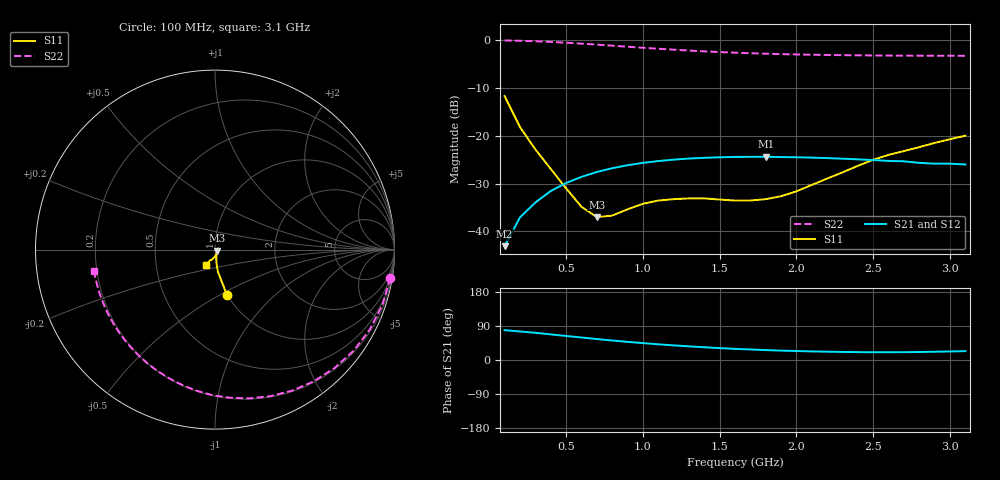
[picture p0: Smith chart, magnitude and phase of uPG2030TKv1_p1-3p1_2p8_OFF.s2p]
! NEC Compound Semiconductor Devices Ltd.
! 21.January 2005
! uPG2030TK
! GaAs MMIC (0.1 - 3.1GHz SPDT switch)
! Vcont1=0v Vcont2=2.8v / IN-OUT1 ( OFF )
! OUT2:50ohm termination
#  GHz  S  MA  R  50
!  f  S11  S21  S12  S22
!  GHz  MAG  ANG  MAG  ANG  MAG  ANG  MAG  ANG
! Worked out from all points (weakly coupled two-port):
!   31 points, 100 MHz to 3.1 GHz, reference 50 ohm
!   highest |S21| = -24.41 dB at 1.8 GHz (marker M1); lowest = -43.1 dB at 100 MHz (marker M2)
!   lowest |S11| = -37.0 dB at 700 MHz (marker M3), VSWR 1.03, Z = 51.3 - j0.683 ohm
!   |S11| at or under -10 dB: start of sweep to end of sweep
!   |S22| runs from -3.3 to -0.1 dB; largest |S21 - S12| = 0.001
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0.1  0.26 -75.2  0.007 78.7  0.007 77.8  0.99 -9.2
0.2  0.123 -82.6  0.014 75.3  0.014 75.4  0.982 -18.3
0.3  0.072 -83.7  0.02 71.8  0.02 71.7  0.971 -27.3
0.4  0.045 -80.8  0.0264 67.6  0.0263 67.7  0.956 -36.1
0.5  0.0282 -72.8  0.032 63.4  0.032 63.4  0.9376 -44.7
0.6  0.0181 -55.5  0.0371 59.4  0.0371 59.2  0.9171 -53.2
0.7  0.0141 -28.2  0.0417 55.3  0.0415 55.1  0.8958 -61.3
0.8  0.0146 -4.1  0.0457 51.5  0.0455 51.4  0.8732 -69.2
0.9  0.017 9.5  0.0491 47.9  0.0488 47.8  0.8514 -76.8
1  0.0194 15.3  0.052 44.6  0.0516 44.3  0.8299 -84.2
1.1  0.021 16.2  0.0543 41.4  0.0541 41.4  0.8113 -91.0
1.2  0.0217 14.1  0.0562 38.6  0.056 38.6  0.7931 -97.5
1.4  0.0221 3.2  0.0587 33.6  0.0585 33.5  0.7612 -109.7
1.6  0.021 -14.0  0.06 29.4  0.0599 29.3  0.7376 -120.5
1.7  0.021 -26.8  0.0601 27.8  0.0599 27.7  0.7282 -125.4
1.8  0.0217 -41.1  0.0602 26.1  0.0598 26.1  0.7197 -130.0
1.9  0.0233 -54.4  0.0598 24.8  0.0596 24.8  0.7128 -134.3
2  0.0262 -65.8  0.0595 23.7  0.0593 23.8  0.7069 -138.4
2.1  0.0306 -77.3  0.059 22.7  0.0588 22.8  0.7024 -142.2
2.5  0.0561 -106.1  0.0556 20.5  0.0555 20.6  0.6899 -155.1
2.6  0.063 -111.5  0.0545 20.6  0.0544 20.6  0.6883 -157.9
3.1  0.1 -121.2  0.05 23.4  0.05 23.4  0.684 -169.8
